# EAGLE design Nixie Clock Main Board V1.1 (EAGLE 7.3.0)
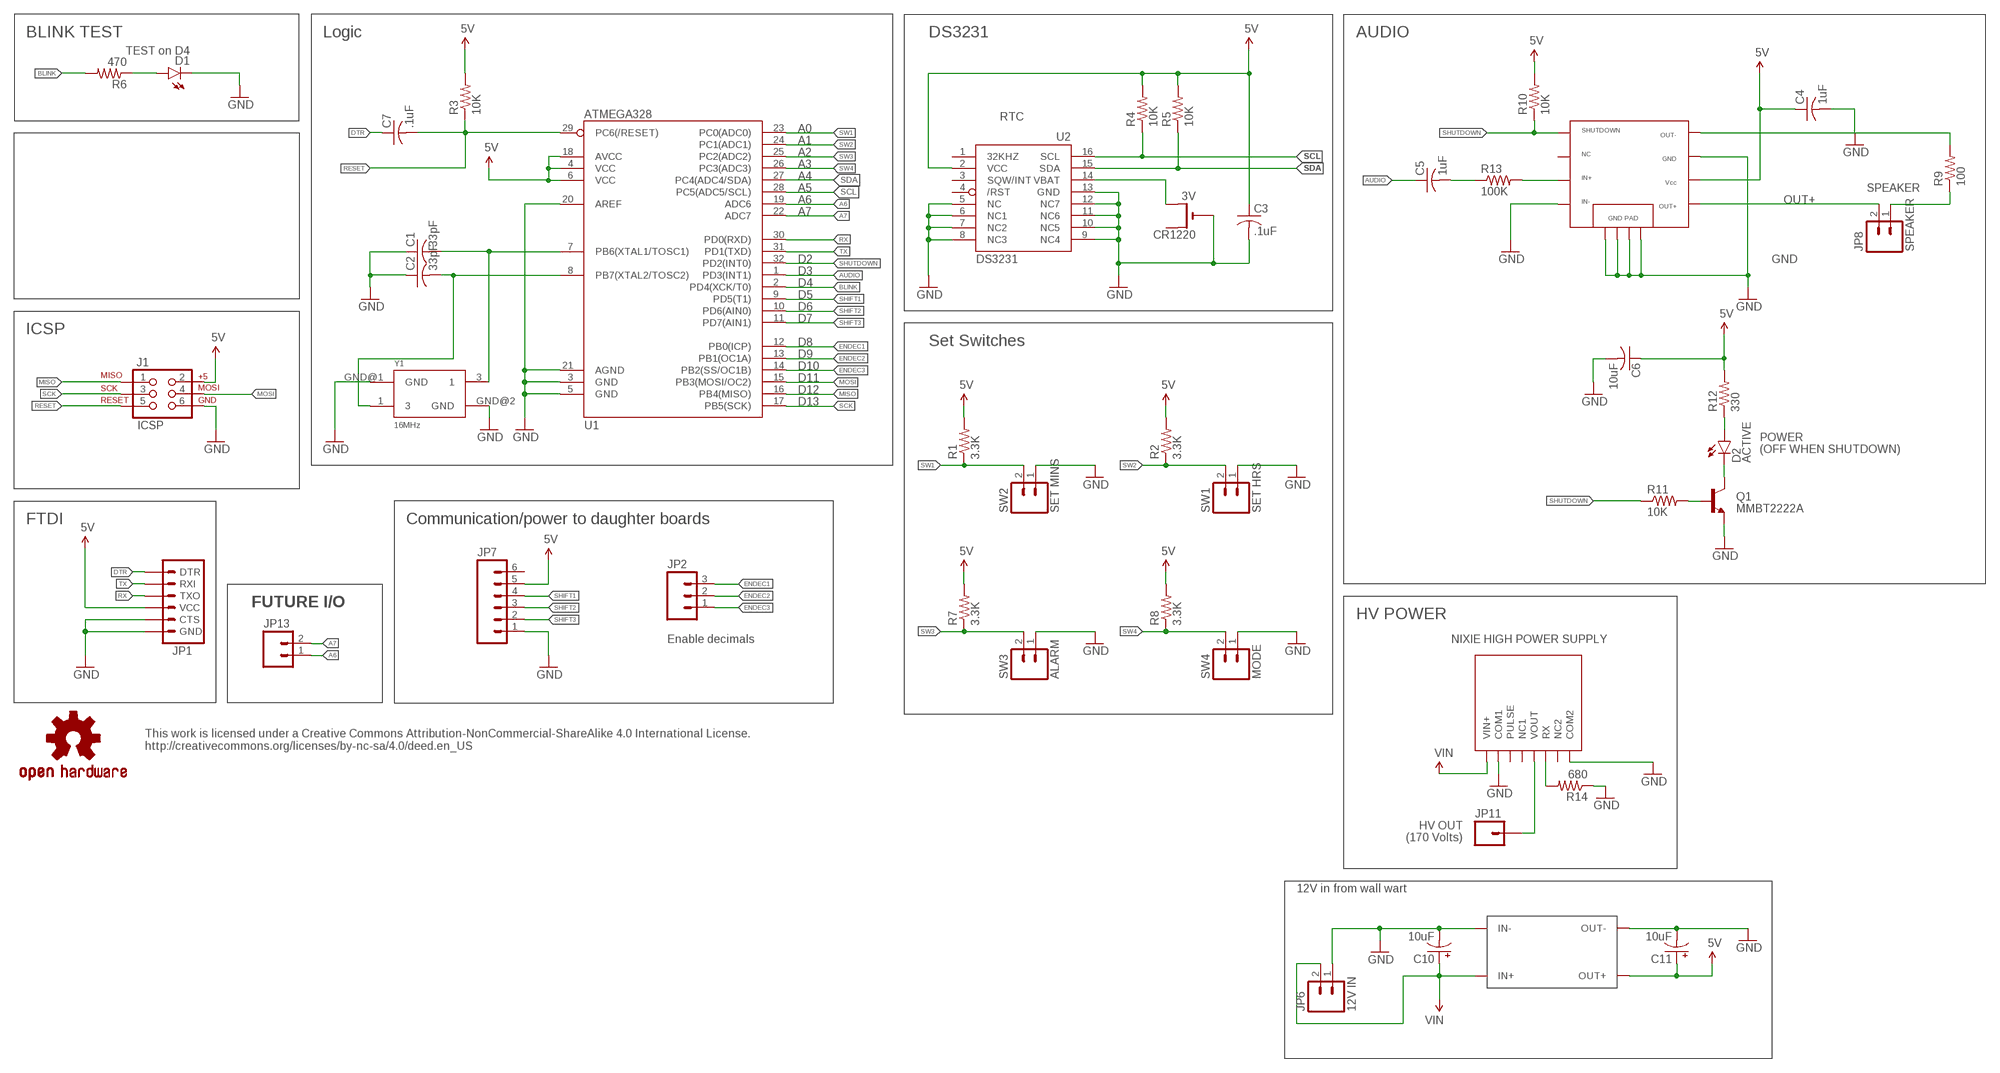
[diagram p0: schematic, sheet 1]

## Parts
C1  33pF  C-USC0805K  [C0805K]
C2  33pF  C-USC0805K  [C0805K]
C3  .1uF  C-USC0805K  [C0805K]
C4  1uF  C-USC0805  [C0805]
C5  1uF  C-USC0805  [C0805]
C6  10uF  C-USC0805  [C0805]
C7  .1uF  C-USC0805K  [C0805K]
C10  10uF  CAP_POLPTH2  [CPOL-RADIAL-10UF-25V]
C11  10uF  CAP_POLPTH2  [CPOL-RADIAL-10UF-25V]
CR1220  3V  CR1220THM  [CR1220-THM]
D1  TEST on D4  LED-RED1206  [LED-1206]
D2  ACTIVE  LED-RED1206  [LED-1206]
J1  ICSP  AVR_SPI_PRG_6PTH  [2X3]
JP1  ARDUINO_SERIAL_PROGRAMSMD  [1X06-SMD]
JP2  M03PTH  [1X03]
JP6  12V IN  M02JST-PTH-2  [JST-2-PTH]
JP7  M06NO_SILK_FEMALE_PTH  [1X06_NO_SILK]
JP8  SPEAKER  M02PTH  [1X02]
JP11  M01  [1X01HV]
JP13  M02PTH  [1X02]
Q1  MMBT2222A  TRANSISTOR_NPNSOT23-3  [SOT23-3]
R1  3.3K  R-US_R0805  [R0805]
R2  3.3K  R-US_R0805  [R0805]
R3  10K  R-US_R0805  [R0805]
R4  10K  R-US_R0805  [R0805]
R5  10K  R-US_R0805  [R0805]
R6  470  R-US_R0805  [R0805]
R7  3.3K  R-US_R0805  [R0805]
R8  3.3K  R-US_R0805  [R0805]
R9  100  R-US_R0805  [R0805]
R10  10K  R-US_R0805  [R0805]
R11  10K  R-US_R0805  [R0805]
R12  330  R-US_R0805  [R0805]
R13  100K  R-US_R0805  [R0805]
R14  680  RESISTORPTH-1/2W  [AXIAL-0.5]
SW1  SET HRS  M02JST-PTH-2  [JST-2-PTH]
SW2  SET MINS  M02JST-PTH-2  [JST-2-PTH]
SW3  ALARM  M02JST-PTH-2  [JST-2-PTH]
SW4  MODE  M02JST-PTH-2  [JST-2-PTH]
U1  ATMEGA328  ATMEGA328_SMT  [TQFP32-08]
U2  DS3231  DS3231/SO  [SO16W]
U3  TPA2005  [MSOP8]
U$2  OSHW-LOGOM  [OSHW-LOGO-M]
U$7  NIXIEPOWERSUPPLY  [NIXIEPWR]
U$10  DCTODC  [DCTODC]
Y1  16MHz  OSCILLATOR5X3  [CRYSTAL-SMD-5X3]

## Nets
5V: C3.1 C4.1 C6.1 C11.1(+) J1.2 JP1.4(VCC) JP7.5 R1.2 R2.2 R3.2 R4.2 R5.2 R7.2 R8.2 R10.2 R12.2 U1.4(VCC) U1.6(VCC) U1.18(AVCC) U2.2(VCC) U3.6 U$10.OUT+
A6: JP13.1 U1.19(ADC6)
A7: JP13.2 U1.22(ADC7)
AUDIO: C5.1 U1.1(PD3(INT1))
BLINK: R6.2 U1.2(PD4(XCK/T0))
DTR: C7.1 JP1.1(DTR)
ENDEC1: JP2.3 U1.12(PB0(ICP))
ENDEC2: JP2.2 U1.13(PB1(OC1A))
ENDEC3: JP2.1 U1.14(PB2(SS/OC1B))
GND: C1.1 C2.1 C3.2 C4.2 C6.2 C10.2(-) C11.2(-) CR1220.- D1.C J1.6 JP1.5(CTS) JP1.6(GND) JP6.1 JP7.1 Q1.2(E) R14.P$1 SW1.1 SW2.1 SW3.1 SW4.1 U1.3(GND) U1.5(GND) U1.20(AREF) U1.21(AGND) U2.5(NC) U2.6(NC1) U2.7(NC2) U2.8(NC3) U2.9(NC4) U2.10(NC5) U2.11(NC6) U2.12(NC7) U2.13(GND) U3.2 U3.4 U3.7 U3.9 U3.10 U3.11 U3.A U3.B U3.C U3.D U$7.P$2(COM1) U$7.P$8(COM2) U$10.IN- U$10.OUT- Y1.GND@1(GND) Y1.GND@2(GND)
HVO: JP11.1 U$7.P$5(VOUT)
IN+AMP: R13.2 U3.3
MISO: J1.1 U1.16(PB4(MISO))
MOSI: J1.4 U1.15(PB3(MOSI/OC2))
N$1: CR1220.+2(+1) U2.14(VBAT)
N$2: D1.A R6.1
N$3: JP8.1 R9.1
N$4: R14.P$2 U$7.P$6(RX)
N$20: R9.2 U3.8
N$25: D2.A R12.1
N$26: Q1.1(B) R11.2
N$27: D2.C Q1.3(C)
N$28: C5.2 R13.1
N$30: C1.2 U1.7(PB6(XTAL1/TOSC1)) Y1.3
N$31: C2.2 U1.8(PB7(XTAL2/TOSC2)) Y1.1
OUT+: JP8.2 U3.5
RESET: C7.2 J1.5 R3.1 U1.29(PC6(/RESET))
RX: JP1.3(TXO) U1.30(PD0(RXD))
SCK: J1.3 U1.17(PB5(SCK))
SCL: R4.1 U1.28(PC5(ADC5/SCL)) U2.16(SCL)
SDA: R5.1 U1.27(PC4(ADC4/SDA)) U2.15(SDA)
SHIFT1: JP7.4 U1.9(PD5(T1))
SHIFT2: JP7.3 U1.10(PD6(AIN0))
SHIFT3: JP7.2 U1.11(PD7(AIN1))
SHUTDOWN: R10.1 R11.1 U1.32(PD2(INT0)) U3.1
SW1: R1.1 SW2.2 U1.23(PC0(ADC0))
SW2: R2.1 SW1.2 U1.24(PC1(ADC1))
SW3: R7.1 SW3.2 U1.25(PC2(ADC2))
SW4: R8.1 SW4.2 U1.26(PC3(ADC3))
TX: JP1.2(RXI) U1.31(PD1(TXD))
VIN: C10.1(+) JP6.2 U$7.P$1(VIN+) U$10.IN+
Unconnected: CR1220.+1(+) JP7.6 U2.1(32KHZ) U2.3(SQW/INT) U2.4(/RST) U3.NC U$7.P$3(PULSE) U$7.P$4(NC1) U$7.P$7(NC2)

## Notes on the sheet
- BLINK TEST | Logic | DS3231 | AUDIO
- RTC
- A0
- A1
- A2
- A3
- A4
- A5 | SPEAKER
- A6
- A7
- D2
- D3
- D4
- D5
- D6
- D7
- ICSP
- D8 | Set Switches
- D9
- D10
- D11
- D12
- D13
- POWER
- (OFF WHEN SHUTDOWN)
- FTDI | Communication/power to daughter boards
- FUTURE I/O
- HV POWER
- Enable decimals | NIXIE HIGH POWER SUPPLY
- This work is licensed under a Creative Commons Attribution-NonCommercial-ShareAlike 4.0 International License.
  http://creativecommons.org/licenses/by-nc-sa/4.0/deed.en_US
- HV OUT
- (170 Volts)
- 12V in from wall wart

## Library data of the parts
C1-C7 = adafruit:C-US: CAPACITOR, American symbol
C10 C11 = SparkFun-Capacitors:CAP_POL: Capacitor Polarized
CR1220 = adafruit:CR1220: CR1216/CR1220/CR1225 12mm 3V lithium coin cell Great for battery packup. Both SMT and THM holders. Note the THM package has the ground pads on both sides of the PCB so that the masks are the same - this reduces the cost
D1 D2 = SparkFun-LED:LED-RED: Assorted Red LEDs; PROD_ID: DIO-00809; VALUE: RED
J1 = SparkFun:AVR_SPI_PRG_6: AVR ISP 6 Pin This is the reduced ISP connector for AVR programming. Common on Arduino. This footprint will take up less PCB space and can be used with a 10-pin to 6-pin adapter such as SKU: BOB-08508; OC_NEWARK: unknown
JP1 = SparkFun-Connectors:ARDUINO_SERIAL_PROGRAM: FTDI connector footprints; PROD_ID: CONN-08971
JP2 = SparkFun-Connectors:M03: Header 3 Standard 3-pin 0.1" header. Use with straight break away headers (SKU : PRT-00116), right angle break away headers (PRT-00553), swiss pins (PRT-00743), machine pins (PRT-00117), and female headers (PRT-00115). Molex polarized connector foot print use with SKU : PRT-08232 with associated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
JP6 SW1-SW4 = SparkFun-Connectors:M02: Standard 2-pin 0.1" header. Use with; PROD_ID: CONN-09863; SKU: PRT-09914
JP7 = SparkFun-Connectors:M06: Header 6 Standard 6-pin 0.1" header. Use with straight break away headers (SKU : PRT-00116), right angle break away headers (PRT-00553), swiss pins (PRT-00743), machine pins (PRT-00117), and female headers (PRT-00115). Molex polarized connector foot print use with SKU : PRT-08094 with associated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; PROD_ID: CONN-08437
JP8 JP13 = SparkFun-Connectors:M02: Standard 2-pin 0.1" header. Use with
JP11 = SparkFun-Connectors:M01: Header 1
Q1 = SparkFun:TRANSISTOR_NPN: Transistor NPN BJT configuration in SOT23 package. MMBT2222 is the common NPN we use. Double check BCE configuration again layout.
R1-R13 = adafruit:R-US_: RESISTOR, American symbol
R14 = SparkFun-Resistors:RESISTOR: Resistor
U1 = SparkFun-DigitalIC:ATMEGA328_SMT: 32-Pin Atmega328 part Commonly used on Arduino compatible boards Available in QFP and QFN packages TQFP is IC-09069 QFN is non-stock; PROD_ID: IC-09069; VALUE: ATMEGA328P
U2 = adafruit:DS3231
U3 = TPA2005:TPA2005
U$2 = SparkFun:OSHW-LOGO: Open Source Hardware Logo This logo indicates the piece of hardware it is found on incorporates a OSHW license and/or adheres to the definition of open source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
U$7 = NixiePowerSupply:NIXIEPOWERSUPPLY
U$10 = DC to DC:DCTODC
Y1 = SparkFun-FreqCtrl:OSCILLATOR: Generic 5x3 and 7x5 oscillators

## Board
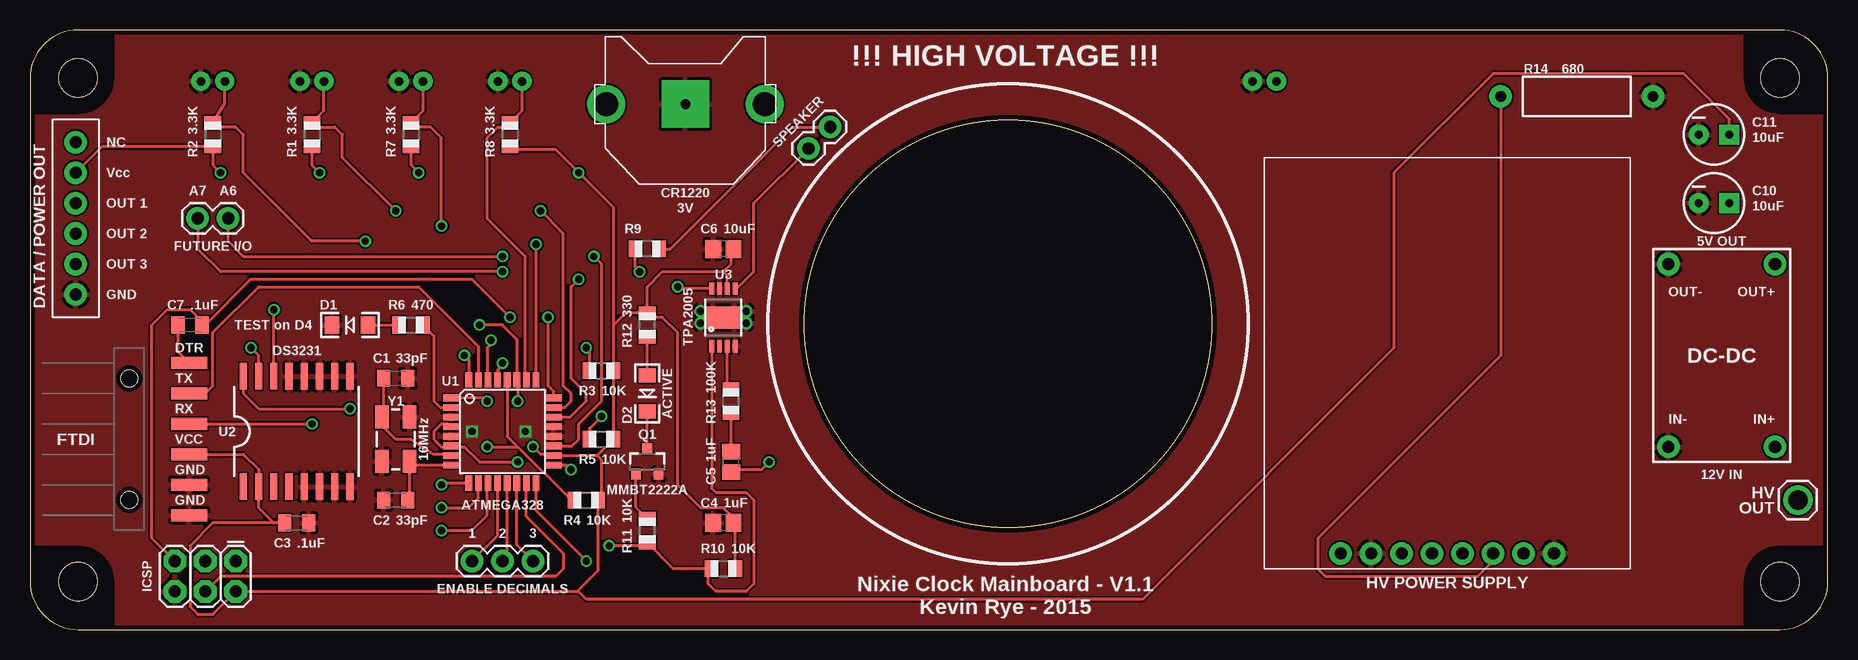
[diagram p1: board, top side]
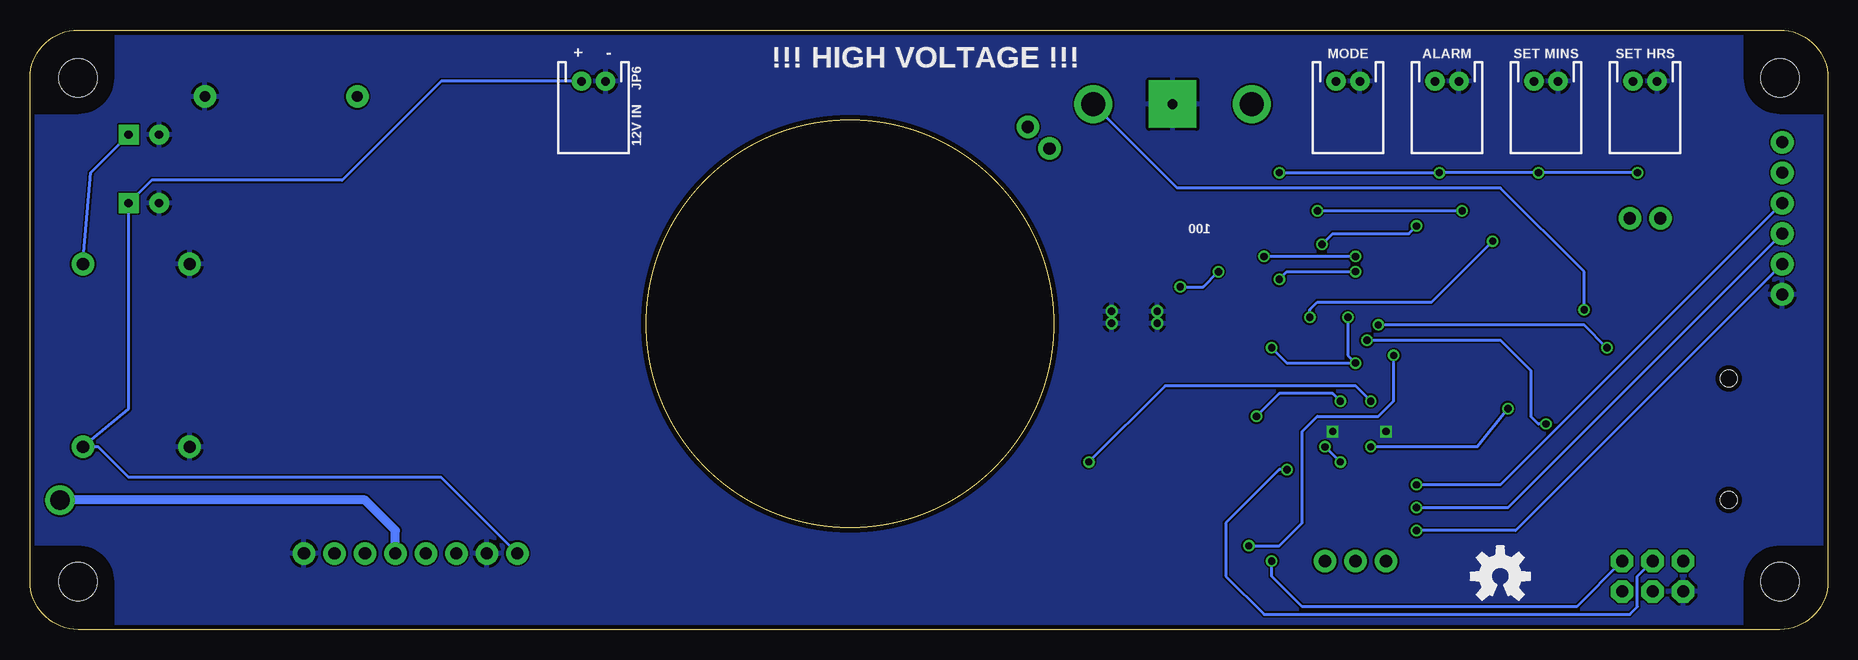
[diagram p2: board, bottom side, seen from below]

Size 149.83 x 50 mm. Coordinates in mm from the lower left corner, seen from the top.
Outline: circle at 81.5,25.5 radius 17
Copper layers (1*16): Top 0.0356mm / dielectric 1.5011mm / Bottom 0.0356mm
Design rules "LaenPCBOrder": minimum track width 6mil, minimum drill 13mil, track to track 6mil, track to pad 6mil, pad to pad 6mil, via to via 6mil, smd to smd 6mil, copper to edge 15mil, drill to drill 6mil, minimum pad ring 7mil, minimum via ring 7mil, stop-mask expansion 3mil, vias tented up to drill 0mil, thermal gap 10mil

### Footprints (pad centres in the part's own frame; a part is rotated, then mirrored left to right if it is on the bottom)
C0805K = smd 1.1 x 1.4: 1 -1,0; 2 1,0
C0805 = smd 1.3 x 1.5: 1 -0.85,0; 2 0.85,0
CPOL-RADIAL-10UF-25V = drill 0.7 pad 1.651 square: 1 1.27,0 | drill 0.7 pad 1.651: 2 -1.27,0
CR1220-THM = drill 2 pad 3.175: +1 -6.604,0; +2 6.604,0 | drill 0.8 pad 3.962 square: - 0,0
LED-1206 = smd 1.2 x 1.4: A -1.5,0; C 1.5,0
2X3 = drill 1.016 pad 1.88 octagon: 1 0,0; 2 0,2.54; 3 2.54,0; 4 2.54,2.54; 5 5.08,0; 6 5.08,2.54
1X06-SMD = smd 1 x 3: 1 -6.35,5; 2 -3.81,5; 3 -1.27,5; 4 1.27,5; 5 3.81,5; 6 6.35,5 | hole 1.4: -5.08,0; 5.08,0
1X03 = drill 1.016 pad 1.88: 1 0,0; 2 2.54,0; 3 5.08,0
JST-2-PTH = drill 0.7 pad 1.6: 1 -1,0; 2 1,0
1X06_NO_SILK = drill 1.016 pad 1.88: 1 0,0; 2 2.54,0; 3 5.08,0; 4 7.62,0; 5 10.16,0; 6 12.7,0
1X02 = drill 1.016 pad 1.88: 1 0,0; 2 2.54,0
1X01HV = drill 1.628 pad 2.464: 1 0,0
SOT23-3 = smd 0.8 x 0.9: 1 -0.95,-1; 2 0.95,-1; 3 0,1.1
R0805 = smd 1.1 x 1.4: 1 -1,0; 2 1,0
AXIAL-0.5 = drill 0.9 pad 1.88: P$1 -6.35,0; P$2 6.35,0
TQFP32-08 = smd 1.27 x 0.559: 1 -4.293,2.8; 2 -4.293,2; 3 -4.293,1.2; 4 -4.293,0.4; 5 -4.293,-0.4; 6 -4.293,-1.2; 7 -4.293,-2; 8 -4.293,-2.8; 17 4.293,-2.8; 18 4.293,-2; 19 4.293,-1.2; 20 4.293,-0.4; 21 4.293,0.4; 22 4.293,1.2; 23 4.293,2; 24 4.293,2.8 | smd 0.559 x 1.27: 9 -2.8,-4.293; 10 -2,-4.293; 11 -1.2,-4.293; 12 -0.4,-4.293; 13 0.4,-4.293; 14 1.2,-4.293; 15 2,-4.293; 16 2.8,-4.293; 25 2.8,4.293; 26 2,4.293; 27 1.2,4.293; 28 0.4,4.293; 29 -0.4,4.293; 30 -1.2,4.293; 31 -2,4.293; 32 -2.8,4.293
SO16W = smd 0.6 x 2.2: 1 -4.445,-4.6; 2 -3.175,-4.6; 3 -1.905,-4.6; 4 -0.635,-4.6; 5 0.635,-4.6; 6 1.905,-4.6; 7 3.175,-4.6; 8 4.445,-4.6; 9 4.445,4.6; 10 3.175,4.6; 11 1.905,4.6; 12 0.635,4.6; 13 -0.635,4.6; 14 -1.905,4.6; 15 -3.175,4.6; 16 -4.445,4.6
MSOP8 = smd 0.41 x 1.02: 1 -0.975,-2.4; 3 0.325,-2.4; 4 0.975,-2.4; 5 0.975,2.4; 6 0.325,2.4; 7 -0.325,2.4; 8 -0.975,2.4; NC -0.325,-2.4 | smd 1.778 x 0.914: 2 -0.889,0.457; 9 -0.889,-0.457; 10 0.889,-0.457; 11 0.889,0.457 | drill 0.61 pad 1.016: A -1.9,-0.5; B 1.91,-0.5; C 1.91,0.5; D -1.9,0.5
50X150 = hole 3.2: 4,4; 145.83,4; 145.83,46; 4,46
NIXIEPWR = drill 1.016 pad 1.88: P$1 6.35,2.54; P$2 8.89,2.54; P$3 11.43,2.54; P$4 13.97,2.54; P$5 16.51,2.54; P$6 19.05,2.54; P$7 21.59,2.54; P$8 24.13,2.54
DCTODC = drill 1.016 pad 1.88: IN+ 10.16,1.27; IN- 1.27,1.27; OUT+ 10.16,16.51; OUT- 1.27,16.51
CRYSTAL-SMD-5X3 = smd 1.9 x 1.1: 1 -1.85,-1.15; 3 1.85,1.15; GND@1 -1.85,1.15; GND@2 1.85,-1.15

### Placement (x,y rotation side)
C1  30.48,20.95 180 top
C2  30.48,10.79 0 top
C3  22.23,8.89 0 top
C4  57.78,8.89 180 top
C5  58.42,13.97 90 top
C6  57.78,31.75 180 top
C7  13.34,25.4 0 top
C10  140.34,35.56 0 top
C11  140.34,41.27 0 top
CR1220  54.61,43.81 0 top
D1  26.67,25.4 180 top
D2  51.44,19.68 270 top
J1  17.14,5.71 180 top
JP1  8.26,15.88 270 top
JP2  41.91,5.71 180 top
JP6  102.87,45.72 180 bottom
JP7  3.81,27.94 90 top
JP8  66.67,41.91 225 top
JP11  147.32,10.79 0 top
JP13  16.51,34.29 180 top
Q1  51.44,13.97 0 top
R1  23.5,41.27 270 top
R2  15.24,41.27 270 top
R3  47.62,21.59 0 top
R4  46.35,10.79 0 top
R5  47.62,15.88 0 top
R6  31.75,25.4 0 top
R7  31.75,41.27 270 top
R8  40.01,41.27 270 top
R9  51.44,31.75 180 top
R10  57.78,5.08 0 top
R11  51.44,8.26 90 top
R12  51.44,25.4 90 top
R13  58.42,19.05 90 top
R14  128.91,44.45 180 top
SW1  15.24,45.72 180 bottom
SW2  23.5,45.72 180 bottom
SW3  31.75,45.72 180 bottom
SW4  40.01,45.72 180 bottom
U1  39.37,16.51 0 top
U2  22.23,16.51 0 top
U3  57.78,26.04 0 top
U$2  27.3,4.45 0 bottom
U$3  [50X150]  0,0 0 top
U$7  102.87,3.81 0 top
U$10  135.25,13.97 0 top
Y1  30.48,15.88 90 top

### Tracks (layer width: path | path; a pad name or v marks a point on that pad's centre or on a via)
5V  (via drill 0.6)
  Top 0.254: JP1.4 17.78,14.61 19.05,13.34 U2.2 19.05,10.16 20.32,8.89 C3.1 15.24,8.89 13.34,6.99 13.34,1.91 13.97,1.27 15.24,1.27 J1.2 45.59,3.17 45.66,3.24 | v32.38,38.1 31.75,38.73 R7.2 | v15.88,38.1 15.24,38.73 R2.2 5.99,40.27 JP7.5 | 48.62,25.4 R3.2 R5.2 47.26,14.51 | 48.62,25.4 48.62,35.2 v45.72,38.1 43.81,40.01 40.27,40.01 R8.2 | 47.26,14.51 U1.18 43.57,14.61 42.55,14.61 v41.91,15.24 | 47.26,14.51 47.62,14.14 47.62,11.06 R4.2 47.35,4.94 45.66,3.24 | U1.4 34.84,17.14 34.29,17.14 33.66,16.51 33.66,15.88 34.29,15.24 35.01,15.24 arc90 U1.6 35.15,15.24 36.2,15.24 37.47,13.97 v40.64,13.97 | R1.2 23.5,38.73 v24.13,38.1 | 45.66,3.24 46.35,2.54 92.71,2.54 113.67,23.5 113.67,38.1 121.92,46.35 137.79,46.35 141.6,42.55 C11.1 | R12.2 51.44,28.57 52.7,29.84 57.78,29.84 | 57.78,29.84 58.42,30.48 58.42,31.54 C6.1 | U3.6 58.11,29.52 57.78,29.84 | R12.2 49.62,26.4 48.62,25.4 | R10.2 58.78,8.74 C4.1 58.63,9.31 57.78,10.16 55.88,10.16 53.98,12.06 53.98,24.77 52.7,26.04 51.8,26.04 R12.2
  Bottom 0.254: v45.72,38.1 v32.38,38.1 v24.13,38.1 v15.88,38.1 | v41.91,15.24 v40.64,13.97 | U$10.OUT+ 144.78,38.1 C11.1
A6  (via drill 0.6)
  Top 0.254: U1.19 45.16,15.31 45.72,15.88 45.72,17.14 47.62,19.05 47.62,30.48 v46.99,31.11 | v39.37,31.11 17.78,31.11 16.51,32.38 JP13.1
  Bottom 0.254: v39.37,31.11 v46.99,31.11
A7  (via drill 0.6)
  Top 0.254: U1.22 45.02,17.71 46.35,19.05 46.35,19.68 45.09,20.95 45.09,28.57 v45.72,29.21 | v39.37,29.84 15.88,29.84 13.97,31.75 JP13.2
  Bottom 0.254: v45.72,29.21 45.09,29.84 v39.37,29.84
AUDIO  (via drill 0.6)
  Top 0.254: C5.1 58.63,13.34 60.96,13.34 v61.59,13.97 | v38.1,19.05 37.84,19.31 U1.1
  Bottom 0.254: v61.59,13.97 55.24,20.32 39.37,20.32 v38.1,19.05
BLINK
  Top 0.254: U1.2 34.2,18.51 33.66,19.05 33.66,24.5 R6.2
DTR
  Top 0.254: JP1.1 12.34,23.14 C7.1
ENDEC1
  Top 0.254: JP2.3 38.97,7.86 U1.12
ENDEC2
  Top 0.254: JP2.2 39.77,6.12 U1.13
ENDEC3
  Top 0.254: JP2.1 40.57,7.05 U1.14
GND  (via drill 0.6)
  other vias: 41.27,16.51 36.83,16.51
  pour Bottom: -0.64,50.8 150.5,50.8 150.5,-0.64 -0.64,-0.64
  pour Top: -1.27,51.44 151.13,51.44 151.13,-1.27 -1.27,-1.27
HVO
  Bottom 0.762: U$7.P$5 119.38,8.26 121.92,10.79 JP11.1
IN+AMP
  Top 0.254: R13.2 58.11,20.36 U3.3
MISO  (via drill 0.6)
  Top 0.254: v46.35,5.71 42.17,9.9 U1.16
  Bottom 0.254: v46.35,5.71 46.35,4.45 43.81,1.91 20.95,1.91 J1.1
MOSI
  Top 0.254: U1.15 41.37,9.43 44.45,6.35 44.45,5.08 43.81,4.45 15.88,4.45 J1.4
N$1  (via drill 0.6)
  Top 0.254: U2.14 v20.32,26.67
  Bottom 0.254: 60.96,43.81 CR1220.+2 54.23,36.83 27.3,36.83 20.32,29.84 v20.32,26.67
N$2
  Top 0.254: D1.A R6.1
N$3
  Top 0.254: R9.1 53.34,31.75 63.5,41.91 JP8.1
N$4
  Top 0.254: R14.P$2 122.56,22.86 107.31,7.62 107.31,5.08 107.95,4.45 120.65,4.45 121.92,5.71 U$7.P$6
N$20  (via drill 0.61 pad 0.69)
  Top 0.254: U3.8 54.12,28.43 v53.98,28.57 | v50.8,29.84 50.44,30.21 R9.2
  Bottom 0.254: v53.98,28.57 52.07,28.57 v50.8,29.84
N$25
  Top 0.254: D2.A R12.1
N$26
  Top 0.254: R11.2 50.48,10.21 Q1.1
N$27
  Top 0.254: Q1.3 D2.C
N$28
  Top 0.254: C5.2 R13.1
N$30
  Top 0.254: U1.7 34.98,14.61 33.66,14.61 31.75,15.88 30.48,15.88 29.33,17.02 Y1.3 29.48,17.88 C1.2
N$31
  Top 0.254: C2.2 31.63,10.95 Y1.1 31.95,13.71 U1.8
OUT+
  Top 0.254: U3.5 58.91,28.43 60.33,29.84 60.33,35.56 JP8.2
RESET  (via drill 0.6)
  Top 0.254: v39.37,22.23 38.97,21.59 U1.29 | v40.01,26.04 36.83,29.21 18.41,29.21 14.61,25.4 C7.2 14.34,25.67 13.34,26.67 11.43,26.67 10.16,25.4 10.16,7.62 J1.5 | R3.1 46.62,23.23 v46.35,23.5
  Bottom 0.254: v46.35,23.5 45.09,22.23 v39.37,22.23 40.01,22.86 v40.01,26.04
RX  (via drill 0.6)
  Top 0.254: JP1.3 v23.5,17.14 | v38.42,24.13 38.42,23.81 38.1,23.5 38.1,20.87 U1.30
  Bottom 0.254: v38.42,24.13 27.3,24.13 24.77,21.59 24.77,17.78 24.13,17.14 v23.5,17.14
SCK  (via drill 0.6)
  Top 0.254: U1.17 44.71,13.71 v45.09,13.34
  Bottom 0.254: v45.09,13.34 45.72,13.34 50.16,8.89 50.16,4.45 46.99,1.27 16.51,1.27 15.88,1.91 15.88,4.45 J1.3
SCL  (via drill 0.6)
  Top 0.254: U1.28 39.77,16.11 40.64,15.24 | 40.64,15.24 45.09,10.79 R4.1 | U2.16 17.78,19.68 19.05,18.41 v26.67,18.41 | v38.1,15.24 40.64,15.24
  Bottom 0.254: v26.67,18.41 29.21,15.24 v38.1,15.24
SDA  (via drill 0.6)
  Top 0.254: U2.15 19.05,22.86 v18.41,23.5 | v40.64,19.05 40.64,20.73 U1.27 40.57,24.2 39.37,25.4 v37.47,25.4 | v47.62,17.78 46.62,16.78 R5.1
  Bottom 0.254: v18.41,23.5 20.32,25.4 v37.47,25.4 | v40.64,19.05 41.27,19.68 45.72,19.68 v47.62,17.78
SHIFT1  (via drill 0.6)
  Top 0.254: v34.29,12.06 34.44,12.22 U1.9
  Bottom 0.254: v34.29,12.06 27.3,12.06 JP7.4
SHIFT2  (via drill 0.6)
  Top 0.254: v34.29,10.16 36.54,10.16 37.37,10.99 U1.10
  Bottom 0.254: v34.29,10.16 26.67,10.16 JP7.3
SHIFT3  (via drill 0.6)
  Top 0.254: v34.29,8.26 36.83,8.26 38.1,9.53 38.1,12.15 U1.11
  Bottom 0.254: v34.29,8.26 26.04,8.26 JP7.2
SHUTDOWN  (via drill 0.6)
  Top 0.254: U3.1 56.81,11.77 57.15,11.43 59.69,11.43 60.33,10.79 60.33,3.81 59.69,3.17 57.15,3.17 56.52,3.81 56.52,4.81 R10.1 53.61,5.08 R11.1 51.16,6.99 v48.26,6.99 | v36.2,22.86 36.57,22.48 U1.32
  Bottom 0.254: v36.2,22.86 36.2,19.05 37.47,17.78 42.55,17.78 43.81,16.51 43.81,8.89 45.72,6.99 v48.26,6.99
SW1  (via drill 0.6)
  Top 0.254: SW2.2 24.5,43.27 R1.1 23.86,41.91 25.4,41.91 26.04,41.27 26.04,39.37 v30.48,34.92 | U1.23 44.55,18.51 45.09,19.05 45.09,19.68 44.45,20.32 44.45,33.02 v42.55,34.92
  Bottom 0.254: v42.55,34.92 v30.48,34.92
SW2  (via drill 0.6)
  Top 0.254: SW1.2 16.24,43.91 R2.1 15.61,41.91 17.14,41.91 17.78,41.27 17.78,38.1 23.5,32.38 v27.94,32.38 | U1.24 43.66,19.84 43.18,20.32 v43.18,26.04
  Bottom 0.254: v43.18,26.04 43.18,26.67 42.55,27.3 33.02,27.3 v27.94,32.38
SW3  (via drill 0.6)
  Top 0.254: SW3.2 32.75,43.27 R7.1 32.12,41.91 33.39,41.91 34.29,41.01 v34.29,33.66 | U1.25 v42.17,32.12
  Bottom 0.254: v42.17,32.12 41.27,33.02 34.92,33.02 v34.29,33.66
SW4
  Top 0.254: R8.1 41.01,43.27 SW4.2 | U1.26 41.27,20.9 41.27,31.11 38.1,34.29 38.1,41.01 39,41.91 39.64,41.91 R8.1 | 39.73,42.27 R8.1
TX
  Top 0.254: JP1.2 14.61,19.68 15.24,20.32 15.24,24.77 19.05,28.57 32.38,28.57 37.37,23.59 U1.31
VIN
  Bottom 0.254: U$7.P$1 115.57,12.7 141.6,12.7 144.15,15.24 U$10.IN+ 141.6,18.41 C10.1 139.7,37.47 123.83,37.47 115.57,45.72 JP6.2

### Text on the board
Unrouted: This work is licensed under a Creative Commons Attribution-NonCommercial-ShareAlike 4.0 International License. / http://creativecommons.org/licenses/by-nc-sa/4.0/deed.en_US
tPlace: !!! HIGH VOLTAGE !!! | NC | Vcc | OUT 1 | DATA / POWER OUT | OUT 2 | FUTURE I/O | OUT 3 | GND | FTDI | HV | OUT | 1 | 2 | 3 | ENABLE DECIMALS
bPlace: - | + | !!! HIGH VOLTAGE !!!
tNames: A7 | A6 | 5V OUT | DTR | DC-DC | TX | RX | VCC | GND | 12V IN | GND | HV POWER SUPPLY | Nixie Clock Mainboard - V1.1 | Kevin Rye - 2015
